(* Logix 5000 AddOnInstructionDefinition export AMCI_NXFE2_Minimum_Registration_Distance; software revision 20.03 *)

ADD_ON_INSTRUCTION AMCI_NXFE2_Minimum_Registration_Distance   (* revision 1.0, vendor AMCI *)
VAR_INPUT
   Minimum_Registration_Distance : DINT; {required}
END_VAR
VAR_IN_OUT
   NXFE2_output_data : _000A:NXFE2_0986AEB4:O:0; {required}
END_VAR
VAR
   command_data_block : INT[10];
        [0]   // Command Bits MSW
        [1]   // Command Bits LSW
        [2]   // Upper Target Position
        [3]   // Lower Target Position
        [4]   // Upper Programmed Speed
        [5]   // Lower Programmed Speed
END_VAR

ROUTINE Logic   (* ladder *)
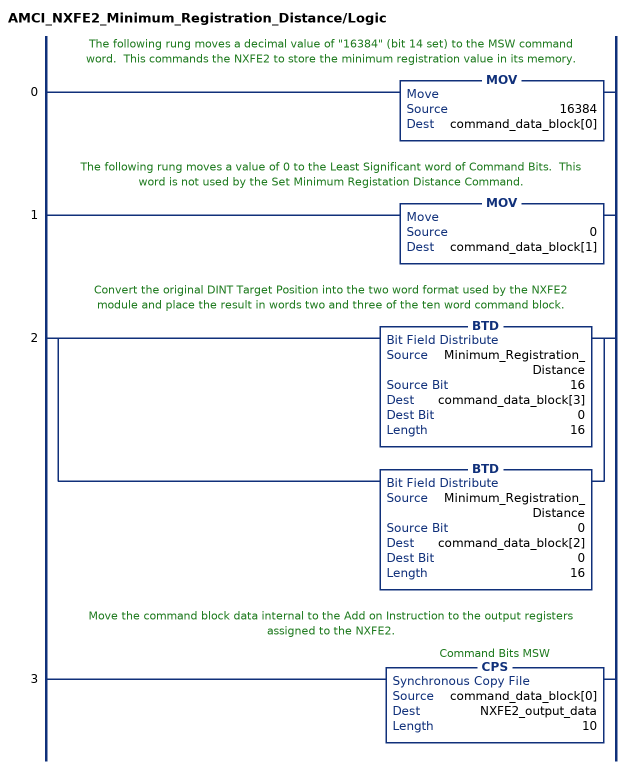
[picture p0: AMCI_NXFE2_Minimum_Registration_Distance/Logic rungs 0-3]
   // The following rung moves a decimal value of "16384" (bit 14 set) to the MSW command word.  This commands the NXFE2 to store the minimum registration value in its memory.
   0: MOV(16384,command_data_block[0]);
   // The following rung moves a value of 0 to the Least Significant word of Command Bits.  This word is not used by the Set Minimum Registation Distance Command.
   1: MOV(0,command_data_block[1]);
   // Convert the original DINT Target Position into the two word format used by the NXFE2 module and place the result in words two and three of the ten word command block.
   2: [BTD(Minimum_Registration_Distance,16,command_data_block[3],0,16) ,BTD(Minimum_Registration_Distance,0,command_data_block[2],0,16) ];
   // Move the command block data internal to the Add on Instruction to the output registers assigned to the NXFE2.
   3: CPS(command_data_block[0],NXFE2_output_data,10);
END_ROUTINE
END_ADD_ON_INSTRUCTION
